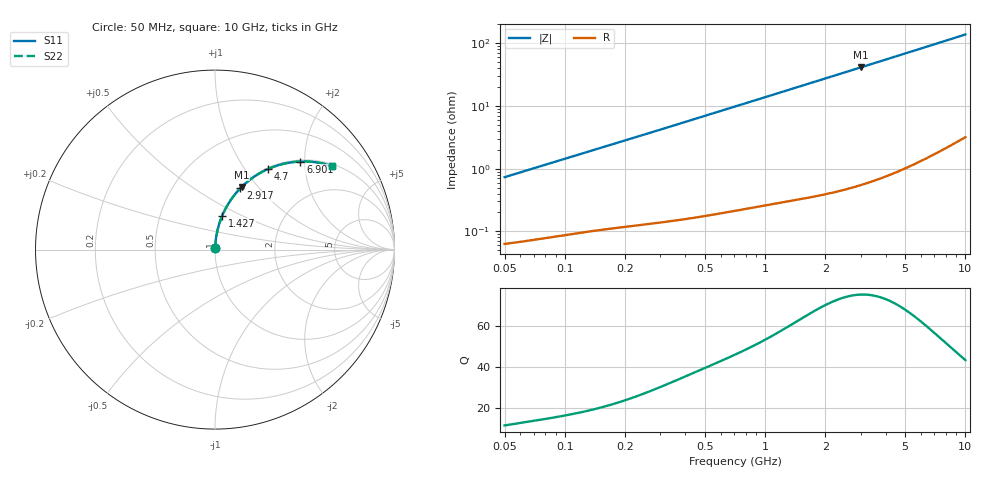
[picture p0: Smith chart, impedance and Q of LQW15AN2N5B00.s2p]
!Murata Part Number: LQW15AN2N5B00
!These Parameters are Measured in Series Mode Connection
!  o--[Z]--o
!Port1  Port2
!  o-------o
!Freq. Start=50[MHz] Stop=10[GHz], 401[Steps]
# Hz S RI R 50
!Freq.(Hz)	S 11(Real)	S 11(Imag)	S 21(Real)	S 21(Imag)	S 12(Real)	S 12(Imag)	S 22(Real)	S 22(Imag)
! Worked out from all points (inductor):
!   401 points, 50 MHz to 10 GHz, reference 50 ohm
!   read as one part in series: L = 2.31 nH near 51.34 MHz
!   highest Q = 75.6 at 2.996 GHz (marker M1), where L = 2.19 nH
!   S11 on the Smith chart (normalised r, x): 50 MHz: 1.00, +0.01; 1.427 GHz: 1.01, +0.39; 2.917 GHz: 1.01, +0.80; 4.7 GHz: 1.02, +1.29; 6.901 GHz: 1.03, +1.90; 10 GHz: 1.06, +2.77
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5e7  0.000682 0.00728  0.9993 -0.00728  0.9993 -0.00728  0.000682 0.00728
5.134228e7  0.000692 0.00747  0.9993 -0.00747  0.9993 -0.00747  0.000692 0.00747
1.214486e8  0.00125 0.0173  0.9987 -0.0173  0.9987 -0.0173  0.00125 0.0173
1.956524e8  0.00192 0.0275  0.9981 -0.0275  0.9981 -0.0275  0.00192 0.0275
2.949953e8  0.00307 0.0411  0.9969 -0.0411  0.9969 -0.0411  0.00307 0.0411
4.689809e8  0.00592 0.0648  0.9941 -0.0648  0.9941 -0.0648  0.00592 0.0648
7.071068e8  0.0116 0.0967  0.9884 -0.0967  0.9884 -0.0967  0.0116 0.0967
1.011124e9  0.0216 0.1364  0.9784 -0.1364  0.9784 -0.1364  0.0216 0.1364
1.426828e9  0.0401 0.1882  0.9599 -0.1882  0.9599 -0.1882  0.0401 0.1882
1.717543e9  0.056 0.2225  0.944 -0.2225  0.944 -0.2225  0.056 0.2225
2.268358e9  0.092 0.2822  0.908 -0.2822  0.908 -0.2822  0.092 0.2822
2.589628e9  0.1159 0.3134  0.8841 -0.3134  0.8841 -0.3134  0.1159 0.3134
2.917498e9  0.142 0.3425  0.858 -0.3425  0.858 -0.3425  0.142 0.3425
2.99582e9  0.1484 0.349  0.8516 -0.349  0.8516 -0.349  0.1484 0.349
3.558764e9  0.1965 0.3907  0.8035 -0.3907  0.8035 -0.3907  0.1965 0.3907
4.171863e9  0.2508 0.4266  0.7492 -0.4266  0.7492 -0.4266  0.2508 0.4266
4.700058e9  0.2976 0.4501  0.7024 -0.4501  0.7024 -0.4501  0.2976 0.4501
5.733131e9  0.3858 0.479  0.6142 -0.479  0.6142 -0.479  0.3858 0.479
6.901252e9  0.4757 0.4908  0.5243 -0.4908  0.5243 -0.4908  0.4757 0.4908
8.198065e9  0.5607 0.4866  0.4393 -0.4866  0.4393 -0.4866  0.5607 0.4866
9.738562e9  0.6422 0.4682  0.3578 -0.4682  0.3578 -0.4682  0.6422 0.4682
1e10  0.6542 0.4643  0.3458 -0.4643  0.3458 -0.4643  0.6542 0.4643
